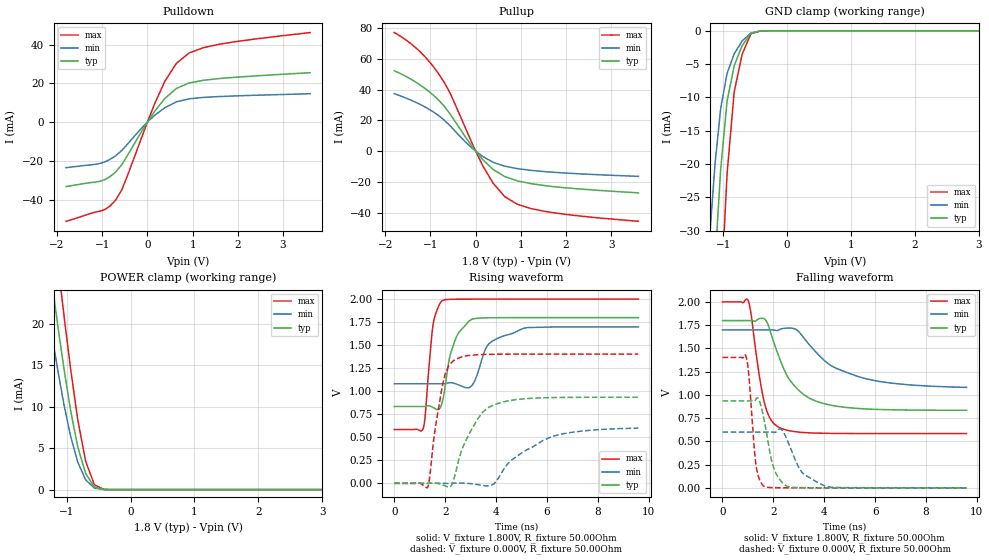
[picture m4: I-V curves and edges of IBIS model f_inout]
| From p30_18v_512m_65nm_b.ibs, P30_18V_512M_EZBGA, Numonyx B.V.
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[Model]   f_inout
Model_type   I/O
Vinl = 0.400V
Vinh = 1.400V
Vmeas = 0.900V
Cref = 30.000pF
|   typ   min   max
C_comp   2.400pF   2.230pF   2.550pF
[Voltage Range]   1.800V   1.700V   2.000V
[Temperature Range]   25.0   85.0   -40.0
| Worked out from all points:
|   slope of the pulldown table from 0 to 0.27 V, typ, clamps not added: 30.4 ohm
|   slope of the pullup table from 0 to 0.27 V, typ, clamps not added: 30.8 ohm
|   GND clamp passes 1 mA (typ) near -0.61 V on its own axis
|   POWER clamp passes 1 mA (typ) near -0.62 V on its own axis
|   falling waveform, V_fixture 1.800V, R_fixture 50.00Ohm: 20-80 % time 1.12ns typ, 1.95ns min, 500ps max; typ from 1.8 V to 0.834 V
|   rising waveform, V_fixture 1.800V, R_fixture 50.00Ohm: 20-80 % time 485ps typ, 782ps min, 267ps max; typ from 0.834 V to 1.8 V
|   rising waveform, V_fixture 0.000V, R_fixture 50.00Ohm: 20-80 % time 938ps typ, 1.73ns min, 468ps max; typ from 0.002 V to 0.934 V
|   falling waveform, V_fixture 0.000V, R_fixture 50.00Ohm: 20-80 % time 428ps typ, 760ps min, 237ps max; typ from 0.934 V to 0.002 V
[Pulldown]
|   Voltage   I(typ)   I(min)   I(max)
-1.8V     -33.3mA    -23.56mA   -51.26mA
-941.4mV  -29.73mA   -20.57mA   -45.18mA
-703.8mV  -25.8mA    -17.43mA   -40.34mA
-563.4mV  -21.9mA    -14.6mA    -34.88mA
-55.8mV   -2.075mA   -1.328mA   -3.457mA
154.8mV   5.4mA      3.379mA    9.181mA
387mV     12.24mA    7.504mA    21.13mA
640.8mV   17.37mA    10.46mA    30.36mA
921.6mV   20.2mA     12.02mA    35.68mA
1.235V    21.6mA     12.76mA    38.43mA
1.575V    22.47mA    13.19mA    40.16mA
3.6V      25.53mA    14.66mA    46.26mA
[GND Clamp]
|   Voltage   I(typ)   I(min)   I(max)
-1.8V     -188.7mA   -146.3mA   -247.7mA
-1.201V   -48.92mA   -29.8mA    -80.44mA
-1.125V   -34.56mA   -19.87mA   -61.24mA
-1.093V   -29.46mA   -16.83mA   -53.63mA
-1.033V   -20.34mA   -11.42mA   -39.86mA
-941.4mV  -10.95mA   -6.591mA   -22.2mA
-936mV    -10.49mA   -6.35mA    -21.29mA
-822.6mV  -5.164mA   -3.397mA   -9.002mA
-703.8mV  -2.26mA    -1.546mA   -3.6mA
-563.4mV  -385.6uA   -320.3uA   -447.6uA
-406.8mV  -9.726uA   -15.31uA   -3.782uA
3.6V      0A         0A         0A
[Pullup]
|   Voltage   I(typ)   I(min)   I(max)
-1.8V     52.29mA    37.38mA    77.1mA
-1.276V   43.99mA    31.1mA     65.95mA
-1.039V   38.92mA    27.37mA    58.7mA
-822.6mV  33.26mA    23.21mA    50.5mA
-563.4mV  24.19mA    16.46mA    37.66mA
-239.4mV  9.836mA    6.442mA    15.96mA
154.8mV   -5.453mA   -3.387mA   -9.344mA
387mV     -11.84mA   -7.201mA   -20.76mA
640.8mV   -16.42mA   -9.734mA   -29.48mA
921.6mV   -19.26mA   -11.33mA   -34.48mA
1.57V     -22.51mA   -13.36mA   -39.31mA
3.6V      -27.06mA   -16.34mA   -45.55mA
[POWER Clamp]
|   Voltage   I(typ)   I(min)   I(max)
-1.8V     61.45mA    49.42mA    76.41mA
-1.341V   31.69mA    24.21mA    41.68mA
-1.309V   29.73mA    22.58mA    39.35mA
-1.206V   23.64mA    17.55mA    32.09mA
-1.098V   17.62mA    12.67mA    24.76mA
-1.066V   15.89mA    11.3mA     22.63mA
-936mV    9.5mA      6.389mA    14.49mA
-822.6mV  5.065mA    3.262mA    8.306mA
-703.8mV  1.98mA     1.211mA    3.465mA
-563.4mV  301.8uA    176.3uA    565.7uA
-406.8mV  9.588uA    6.704uA    13.41uA
3.6V      0A         0A         0A
[Ramp]
R_load = 50.00Ohm
|   typ   min   max
dV/dt_r   559.730mV/937.819ps 358.721mV/1.733ns   840.116mV/467.659ps
dV/dt_f   577.921mV/1.122ns   370.269mV/1.951ns   847.900mV/499.854ps
[Falling Waveform]
V_fixture = 1.800V
V_fixture_min = 1.700V
V_fixture_max = 2.000V
R_fixture = 50.00Ohm
|   Time   V(typ)   V(min)   V(max)
0s        1.797V     1.697V     1.998V
1.01ns    1.797V     1.697V     2.013V
1.63ns    1.819V     1.697V     936.4mV
1.85ns    1.709V     1.697V     757.2mV
2.15ns    1.462V     1.69V      662.4mV
2.72ns    1.132V     1.717V     610.2mV
3.72ns    927.8mV    1.446V     588.9mV
4.47ns    878.7mV    1.285V     585.7mV
5.85ns    846.1mV    1.16V      584.5mV
9.6ns     834.1mV    1.08V      584.4mV
[Rising Waveform]
V_fixture = 1.800V
V_fixture_min = 1.700V
V_fixture_max = 2.000V
R_fixture = 50.00Ohm
|   Time   V(typ)   V(min)   V(max)
0s        834.1mV    1.08V      584.4mV
1.13ns    834mV      1.08V      589mV
1.22ns    835.3mV    1.08V      742.1mV
1.53ns    822.3mV    1.08V      1.726V
1.92ns    919.6mV    1.08V      1.986V
2.38ns    1.542V     1.083V     1.996V
3.06ns    1.781V     1.064V     1.997V
3.7ns     1.796V     1.507V     1.998V
5.07ns    1.797V     1.68V      1.998V
9.6ns     1.797V     1.697V     1.998V
[Rising Waveform]
V_fixture = 0.000V
V_fixture_min = 0.000V
V_fixture_max = 0.000V
R_fixture = 50.00Ohm
|   Time   V(typ)   V(min)   V(max)
0s        1.586mV    1.765mV    1.278mV
1.32ns    1.55mV     1.765mV    -39.79mV
1.93ns    -17.9mV    1.539mV    1.108V
2.23ns    -27.49mV   2.256mV    1.303V
2.45ns    162.2mV    3.631mV    1.35V
3.28ns    698.4mV    -12.8mV    1.395V
3.96ns    856.1mV    7.875mV    1.4V
4.61ns    901.1mV    252.1mV    1.401V
6.2ns     930.5mV    508.6mV    1.401V
9.6ns     934.5mV    599.6mV    1.401V
[Falling Waveform]
V_fixture = 0.000V
V_fixture_min = 0.000V
V_fixture_max = 0.000V
R_fixture = 50.00Ohm
|   Time   V(typ)   V(min)   V(max)
0s        934.5mV    599.6mV    1.401V
930ps     934.5mV    599.6mV    1.408V
1.04ns    934.5mV    599.6mV    1.198V
1.32ns    956.3mV    599.6mV    240.4mV
1.65ns    713.4mV    599.6mV    14.33mV
2.01ns    218.6mV    598.1mV    3.27mV
2.56ns    16mV       504.9mV    1.829mV
3.11ns    3.726mV    174.1mV    1.472mV
4.13ns    2.019mV    14.62mV    1.308mV
9.6ns     1.586mV    1.765mV    1.278mV
